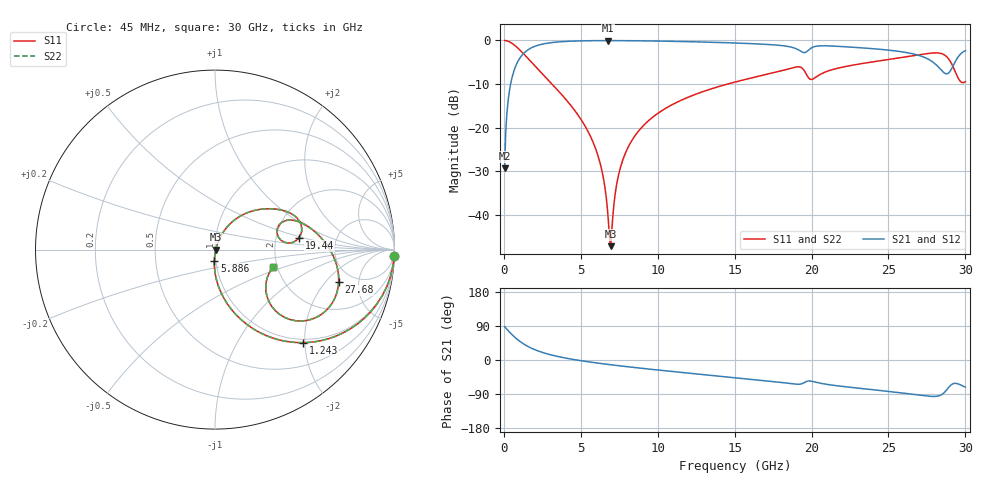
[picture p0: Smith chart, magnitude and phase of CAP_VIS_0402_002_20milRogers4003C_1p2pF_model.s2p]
! S-parameter model data by Modelithics Inc.  support@modelithics.com  813-866-6335  Tampa FL USA
! S-Parameter data specifications:
! Substrate: 20-mil Rogers 4003C, substrate thickness, H=0.508mm, Dielectric constant, Er=3.75
! PCB Mounting Pad Footprint: Pad width, PadW=0.50mm , Pad length, PadL=0.50mm , Pad gap, PadG (edge-to-edge)=0.40mm , Reference planes=1.4mm apart
! Created Wed Nov 18 12:36:28 2015
# hz S ma R 50
! 2 Port Network Data from SP1.SP block
! freq  magS11  angS11  magS21  angS21  magS12  angS12  magS22  angS22
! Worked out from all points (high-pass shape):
!   401 points, 45 MHz to 30 GHz, reference 50 ohm
!   highest |S21| = -0.04 dB at 6.785 GHz (marker M1); lowest = -29.3 dB at 45 MHz (marker M2)
!   |S21| within 3 dB of the highest: 1.264 GHz to 26.55 GHz (25.28 GHz wide, 182 % of centre); 29.71 GHz to end of sweep
!   lowest |S11| = -47.1 dB at 6.935 GHz (marker M3), VSWR 1.01, Z = 50.4 - j0.0332 ohm
!   |S11| at or under -10 dB: 3.132 GHz to 14.53 GHz (11.4 GHz wide, 129 % of centre)
!   |S22| runs from -47.1 to 0.0 dB; largest |S21 - S12| = 0
!   S11 on the Smith chart (normalised r, x): 45 MHz: 1, -56; 1.243 GHz: 0.93, -1.96; 5.886 GHz: 0.99, -0.12; 19.44 GHz: 2.70, +0.45; 27.68 GHz: 3.79, -2.80; 30 GHz: 1.89, -0.42
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4.5e7  0.9994 -2.0  0.03429 88.0  0.03429 88.0  0.9994 -2.0
2.696625e8  0.9794 -12.1  0.2017 77.9  0.2017 77.9  0.9794 -12.1
4.194375e8  0.952 -18.6  0.3056 71.4  0.3056 71.4  0.952 -18.6
1.2432e9  0.7139 -46.6  0.6989 43.3  0.6989 43.3  0.7139 -46.6
2.666062e9  0.3865 -71.7  0.9197 17.9  0.9197 17.9  0.3865 -71.7
5.062462e9  0.1205 -90.5  0.9889 -2.2  0.9889 -2.2  0.1205 -90.5
5.886225e9  0.06235 -93.4  0.9939 -7.0  0.9939 -7.0  0.06235 -93.4
6.410438e9  0.02982 -91.8  0.9952 -9.9  0.9952 -9.9  0.02982 -91.8
6.784875e9  0.00887 -72.8  0.9955 -11.8  0.9955 -11.8  0.00887 -72.8
6.93465e9  0.004399 -4.3  0.9954 -12.5  0.9954 -12.5  0.004399 -4.3
7.383975e9  0.02523 65.0  0.995 -14.7  0.995 -14.7  0.02523 65.0
7.908188e9  0.05168 67.6  0.9938 -17.2  0.9938 -17.2  0.05168 67.6
1.007992e10  0.1491 61.2  0.9832 -26.7  0.9832 -26.7  0.1491 61.2
1.50225e10  0.3337 42.1  0.9347 -46.6  0.9347 -46.6  0.3337 42.1
1.831755e10  0.4632 26.3  0.8617 -60.7  0.8617 -60.7  0.4632 26.3
1.944086e10  0.4722 7.9  0.7299 -61.5  0.7299 -61.5  0.4722 7.9
2.003996e10  0.359 15.9  0.8296 -56.4  0.8296 -56.4  0.359 15.9
2.505742e10  0.6067 4.7  0.7723 -83.2  0.7723 -83.2  0.6067 4.7
2.767849e10  0.7125 -14.8  0.5974 -95.8  0.5974 -95.8  0.7125 -14.8
2.895158e10  0.5998 -41.4  0.4314 -70.5  0.4314 -70.5  0.5998 -41.4
2.947579e10  0.3872 -41.8  0.6273 -62.5  0.6273 -62.5  0.3872 -41.8
3e10  0.3375 -17.1  0.7645 -71.6  0.7645 -71.6  0.3375 -17.1
